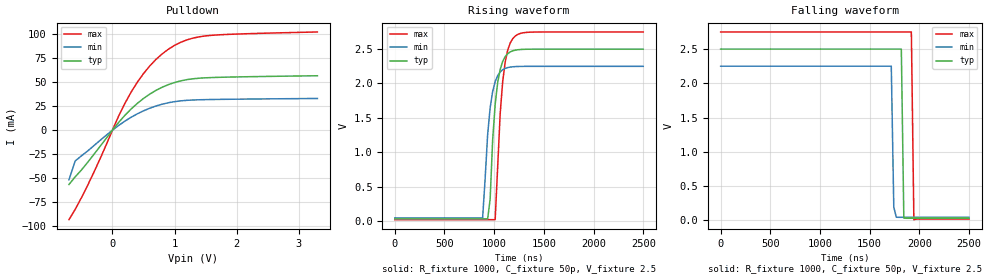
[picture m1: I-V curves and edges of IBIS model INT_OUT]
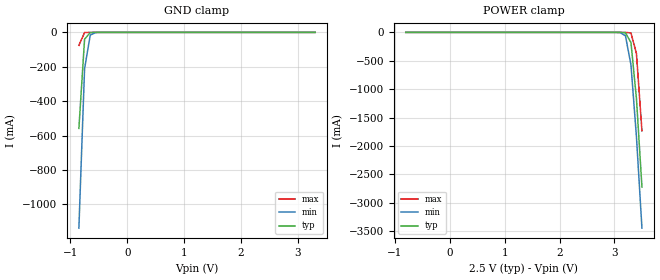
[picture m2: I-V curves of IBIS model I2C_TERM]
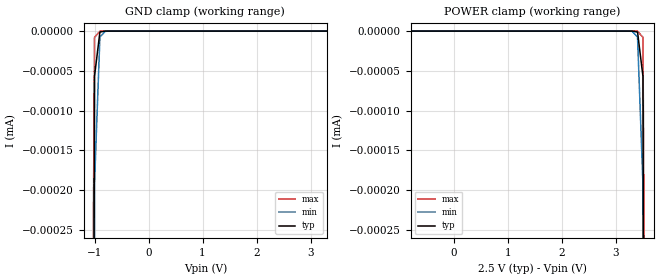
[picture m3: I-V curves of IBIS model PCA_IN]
|   NXP Semiconductors Inc.
|   Specialty Logic Products Group
|   IBIS model of PCA9543C
|   2-Channel I2C switch with
|   interrupt logic and reset
[IBIS Ver]   3.2
[Comment Char]   |_char
| VDD: Typ: 2.5v, Min: 2.25v, 2.75v
[File name]   pca9543c_2_5v.ibs
[File Rev]   1.0
[Date]   Dec 12, 2007 10:55:50 AM
[Source]
Generated by Seshadri Venkataramanan with IbisToolKit at Tempe, AZ
[Notes]
[Disclaimer]
(C) Copyright 2007 NXP Semiconductors
All rights reserved
NXP Semiconductors (NXP) does not warrant that this model and any other
accompanying information (Model) accurately or fully represents the
operating characteristics and specifications of the semiconductor
products to which the Model relates.  Moreover, the Model is furnished
on an "as is" and with "all faults" basis, and without support or
warranty of any kind.  NXP disclaims all warranties, whether expressed
or implied or statutory, including without limitation all implied
warranties of non-infringement, merchantability and fitness for any
purpose, and those arising from a course of dealing or usage of trade.
NXP does not convey any license under its or any third party's patents,
copyrights or other intellectual property or proprietary rights.
You and your company assume any and all risks and liability arising out
of the application or use of the Model.
In no event shall NXP be liable for any direct, indirect, special,
consequential or incidental damages, however caused, whether in
warranty, contract or tort (including negligence), strict liability or
other legal theory, including, without limitation, for lost profits,
business interruption, or corruption or loss of data or information,
arising out of or in connection with the use of or the inability to use
the Model, even if NXP has been advised of the possibility of such
damages.
NXP provides the Model as a courtesy to our customers. You and your
company shall not distribute, convey, sell, or give the Model to anyone
else without receiving prior written permission from NXP.
NXP reserves the right to make changes without notice to the Model to
improve reliability, function, or design.
Please be aware that your receipt and subsequent use of the Model shall
serve as acceptance of these terms and conditions.  If you do not
accept these terms, return or destroy the Model immediately.
[Copyright]
2007
[Component]   PCA9543AD
Si_location Pin
Timing_location Pin
[Manufacturer]   NXP Semiconductors
[Package]
|   variable   typ   min   max
R_pkg   4.54E-02   4.38E-02   5.01E-02
L_pkg   2.31E-09   1.63E-09   3.26E-09
C_pkg   0.565E-12   0.437E-12   0.736E-12
|  SO14
[Pin] signal_name   model_name   R_pin   L_pin   C_pin
1   A0   PCA_IN   4.18E-02  3.26E-09  0.675E-12
2   A1   PCA_IN   5.01E-02  2.30E-09  0.574E-12
3   RESETB   PCA_IN   4.52E-02  1.71E-09  0.467E-12
4   INT0B   INT_IN   4.38E-02  1.63E-09  0.437E-12
5   SD0   I2C_TERM   4.52E-02  1.71E-09  0.465E-12
6   SC0   I2C_TERM   5.01E-02  2.30E-09  0.573E-12
7   VSS   GND   4.18E-02  3.26E-09  0.736E-12
8   INT1B   INT_IN   4.18E-02  3.26E-09  0.736E-12
9   SD1   I2C_TERM   5.01E-02  2.30E-09  0.573E-12
10   SC1   I2C_TERM   4.52E-02  1.71E-09  0.465E-12
11   INTB   INT_OUT   4.38E-02  1.63E-09  0.437E-12
12   SCL   I2C_TERM   4.52E-02  1.71E-09  0.467E-12
13   SDA   I2C_TERM   5.01E-02  2.30E-09  0.574E-12
14   VDD   POWER   4.18E-02  3.26E-09  0.736E-12
[Component]   PCA9543APW
Si_location Pin
Timing_location Pin
[Manufacturer]   NXP Semiconductors
[Package]
|   variable   typ   min   max
R_pkg   3.44E-02   2.80E-02   4.33E-02
L_pkg   1.83E-09   1.36E-09   2.32E-09
C_pkg   0.380E-12   0.302E-12   0.442E-12
|  TSSOP14
[Pin] signal_name   model_name   R_pin   L_pin   C_pin
1   A0   PCA_IN   3.46E-02  2.32E-09  0.423E-12
2   A1   PCA_IN   4.33E-02  2.04E-09  0.441E-12
3   RESETB   PCA_IN   2.80E-02  1.36E-09  0.307E-12
4   INT0B   INT_IN   2.88E-02  1.38E-09  0.302E-12
5   SD0   I2C_TERM   2.80E-02  1.36E-09  0.308E-12
6   SC0   I2C_TERM   4.33E-02  2.04E-09  0.441E-12
7   VSS   GND   3.46E-02  2.32E-09  0.433E-12
8   INT1B   INT_IN   3.46E-02  2.32E-09  0.433E-12
9   SD1   I2C_TERM   4.33E-02  2.04E-09  0.441E-12
10   SC1   I2C_TERM   2.80E-02  1.36E-09  0.308E-12
11   INTB   INT_OUT   2.88E-02  1.38E-09  0.302E-12
12   SCL   I2C_TERM   2.80E-02  1.36E-09  0.308E-12
13   SDA   I2C_TERM   4.33E-02  2.04E-09  0.442E-12
14   VDD   POWER   3.46E-02  2.31E-09  0.433E-12
[Series Pin Mapping] pin_2 model_name   function_table_group
5   13   PCA_SW   1
6   12   PCA_SW   1
9   13   PCA_SW   2
10   12   PCA_SW   2
[Series Switch Groups]
|   Default both off
Off 1 2 /
|  Other possibilities
On 1 /
On 2 /
[Model]   PCA_SW
Model_type Series_switch
C_comp   0.5p   0.5p   0.5p
[Temperature Range] 27   -40   85
[Voltage Range]   3.3   2.3   5.5
[Pullup Reference]  3.3   2.3   5.5
[Pulldown Reference]0   0   0
[On]
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[Off]
|   variable   R(typ)   R(min)   R(max)
[R Series]   1e06   1e06   1e06
|[End   PCA_SW
| Models and submodels in the file (5): INT_OUT (Open_drain), I2C_TERM (Terminator), PCA_IN (Input), INT_IN (Input), PCA_SW (Series_switch)
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[Model]   INT_OUT
Model_type Open_drain
Vref=2.5
Vmeas=1.25
Rref=1000
Cref=1p
C_comp   2.2p   2p   2.3p
[Temperature Range] 27   85   -40
[Voltage Range]   2.5   2.25   2.75
[Pullup Reference]  2.5   2.25   2.75
[Pulldown Reference]0   0   0
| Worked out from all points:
|   slope of the pulldown table from 0 to 0.375 V, typ, clamps not added: 14.2 ohm
|   falling waveform, R_fixture 1000, C_fixture 50p, V_fixture 2.5: 20-80 % time 15.2ns typ, 16.2ns min, 15.1ns max; typ from 2.5 V to 0.029 V
|   rising waveform, R_fixture 1000, C_fixture 50p, V_fixture 2.5: 20-80 % time 69.2ns typ, 73.4ns min, 73.3ns max; typ from 0.029 V to 2.5 V
[Pulldown]
-700mV    -56.73mA   -51.78mA   -93.46mA
-600mV    -48.74mA   -32.17mA   -82.78mA
-300mV    -25.4mA    -16.24mA   -44.15mA
100mV     8.124mA    4.947mA    14.76mA
300mV     22.07mA    13.48mA    39.67mA
500mV     33.12mA    20.21mA    59.1mA
600mV     37.64mA    22.93mA    67.01mA
800mV     44.84mA    27.14mA    79.64mA
1.1V      51.52mA    30.64mA    91.81mA
1.4V      54.31mA    31.77mA    97.55mA
1.9V      55.49mA    32.31mA    100.1mA
3.3V      56.85mA    33.12mA    102.6mA
[Falling Waveform]
R_fixture=1000
C_fixture=50p
V_fixture=2.5
V_fixture_min=2.25
V_fixture_max=2.75
0s        2.5V       2.25V      2.75V
1.717us   2.5V       2.25V      2.75V
1.742us   2.5V       192.2mV    2.75V
1.768us   2.5V       44.1mV     2.75V
1.818us   2.5V       43.56mV    2.75V
1.843us   31.57mV    43.56mV    2.75V
1.919us   29.48mV    43.56mV    2.75V
1.944us   29.48mV    43.56mV    8.562mV
1.97us    29.48mV    43.56mV    17.78mV
2.5us     29.48mV    43.56mV    17.77mV
[Rising Waveform]
R_fixture=1000
C_fixture=50p
V_fixture=2.5
V_fixture_min=2.25
V_fixture_max=2.75
0s        29.47mV    43.53mV    17.77mV
883.8ns   29.47mV    43.54mV    17.78mV
934.3ns   29.48mV    1.257V     17.78mV
959.6ns   322mV      1.647V     17.79mV
1.01us    1.698V     2.028V     17.8mV
1.061us   2.205V     2.168V     1.563V
1.086us   2.321V     2.2V       2.03V
1.136us   2.434V     2.232V     2.486V
1.212us   2.485V     2.246V     2.691V
2.5us     2.5V       2.25V      2.75V
[Ramp]
R_load=1000
dV/dt_r   1.482E+0/9.677E-10   1.471E+0/1.207E-9   1.490E+0/7.549E-10
dV/dt_f   1.482E+0/1.129E-9   1.471E+0/2.120E-9   1.490E+0/6.164E-10
|[End   INT_OUT
| [End   I2C_TERM
[Model]   I2C_TERM
Model_type Terminator
C_comp   9.5p   9.5p   9.5p
[Temperature Range] 27   85   -40
[Voltage Range]   2.5   2.25   2.75
[Pullup Reference]  2.5   2.25   2.75
[Pulldown Reference]0   0   0
[POWER Clamp Reference]2.5   2.25   2.75
[GND Clamp Reference]0   0   0
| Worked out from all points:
|   GND clamp passes 1 mA (typ) near -0.63 V on its own axis
[GND Clamp]
|   -6.000000E-1   -1.554225E-1   -1.242642E-1   -2.666059E-1
|   -5.000000E-1   -1.602113E-1   -1.179351E-1   -2.662641E-1
|   -4.000000E-1   -1.574088E-1   -1.099432E-1   -2.800035E-1
-850mV    -558.2mA   -1.138A    -75.48mA
-750mV    -39.88mA   -211.4mA   -978.6uA
-650mV    -1.319mA   -15.35mA   -6.907uA
-550mV    -28.76uA   -817.5uA   -47.66nA
-450mV    -602.7nA   -33.05uA   -372.7pA
3.3V      259.2pA    288.8pA    267.5pA
[POWER Clamp]
-800mV    259.2pA    288.8pA    267.5pA
3V        -4.164uA   -166.1uA   -4.002nA
3.1V      -197.6uA   -3.751mA   -573.5nA
3.2V      -7.846mA   -59.49mA   -83.04uA
3.3V      -178.6mA   -572mA     -9.962mA
3.4V      -1.167A    -1.838A    -373.6mA
3.5V      -2.722A    -3.446A    -1.735A
[Model]   PCA_IN
Model_type Input
Vinh=2.1
Vinl=0.9
C_comp   1.73p   1.73p   1.73p
[Temperature Range] 27   85   -40
[Voltage Range]   2.5   2.25   2.75
[POWER Clamp Reference]2.5   2.25   2.75
[GND Clamp Reference]0   0   0
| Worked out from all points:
|   GND clamp passes 1 mA (typ) near -1.21 V on its own axis
[GND Clamp]
-2V       -10.17A    -9.093A    -11.52A
-1.1V     -2.718uA   -4.916uA   -1.14uA
-1V       -56.9nA    -192.5nA   -7.858nA
-900mV    -1.192nA   -7.538nA   -55.05pA
-800mV    -25.74pA   -295.9pA   -1.173pA
-700mV    -1.222pA   -12.26pA   -702.6fA
3.3V      3.3pA      3.3pA      3.3pA
[POWER Clamp]
-800mV    3.3pA      3.3pA      3.3pA
3.2V      -1.222pA   -12.26pA   -702.6fA
3.3V      -25.74pA   -295.9pA   -1.173pA
3.4V      -1.192nA   -7.538nA   -55.05pA
3.5V      -56.9nA    -192.5nA   -7.858nA
3.6V      -2.718uA   -4.916uA   -1.14uA
4.5V      -10.17A    -9.093A    -11.52A
